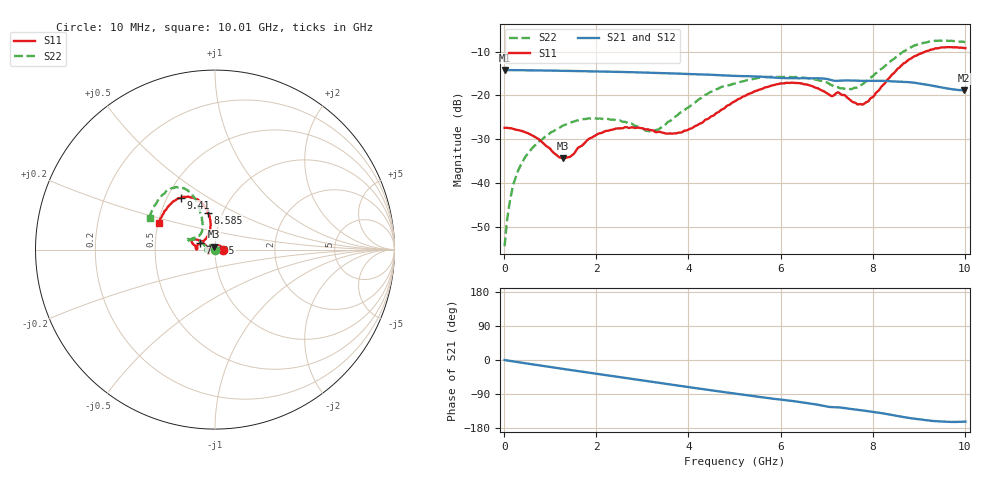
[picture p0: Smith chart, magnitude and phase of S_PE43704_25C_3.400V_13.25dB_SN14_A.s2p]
! Device ID: PE43704
! Dir: z:\PE43704\PE43704_Char_1_20130516\PE43704\AMB\3p400V\13p25dB
! Serial: 14
! Insertion: A
! Impedance: 50 ohm
! Temp: Amb
! VDD: 3.400V
! Attenuation Step: 13.25dB
! IDD: 1.140195e-01mA
#  Hz  S  RI  R  50
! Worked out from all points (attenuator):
!   401 points, 10 MHz to 10.01 GHz, reference 50 ohm
!   highest |S21| = -14.22 dB at 10 MHz (marker M1); lowest = -18.9 dB at 9.985 GHz (marker M2)
!   lowest |S11| = -34.4 dB at 1.285 GHz (marker M3), VSWR 1.04, Z = 49.2 + j1.69 ohm
!   |S11| at or under -10 dB: start of sweep to 9.14 GHz
!   |S22| runs from -54.5 to -7.5 dB; largest |S21 - S12| = 0.0017
!   S11 on the Smith chart (normalised r, x): 10 MHz: 1.09, +0.00; 7.485 GHz: 0.84, +0.06; 8.585 GHz: 0.85, +0.37; 9.41 GHz: 0.59, +0.38; 10.01 GHz: 0.50, +0.17
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1e7  0.0425 0.000286  0.1946 -0.000713  0.1947 -0.00069  0.00183 0.000487
1.6e8  0.0415 0.00618  0.1938 -0.0105  0.1938 -0.0105  0.00161 0.00748
3.6e8  0.037 0.0137  0.1924 -0.023  0.1922 -0.0232  -0.00208 0.0158
7.35e8  0.0222 0.0231  0.187 -0.0454  0.187 -0.0454  -0.0147 0.025
1.285e9  -0.00815 0.0172  0.1747 -0.0764  0.1746 -0.0763  -0.0411 0.0192
1.685e9  -0.0263 0.00321  0.1624 -0.0968  0.1625 -0.0967  -0.0531 0.00531
2.01e9  -0.0346 -0.00853  0.1505 -0.1119  0.1506 -0.1117  -0.0538 -0.00518
2.435e9  -0.0364 -0.0204  0.133 -0.1292  0.1331 -0.1292  -0.0504 -0.0113
3.11e9  -0.0336 -0.0234  0.1013 -0.1507  0.1016 -0.1506  -0.0391 -0.00169
3.36e9  -0.0334 -0.0188  0.0886 -0.1565  0.0888 -0.1564  -0.0405 0.00649
4.01e9  -0.0407 0.00406  0.0548 -0.1663  0.055 -0.1662  -0.0671 0.0303
4.46e9  -0.051 0.022  0.0315 -0.1693  0.0317 -0.1694  -0.0944 0.0528
5.01e9  -0.0741 0.0426  0.00461 -0.1666  0.00472 -0.1668  -0.1257 0.0542
5.96e9  -0.122 0.0575  -0.038 -0.1537  -0.0374 -0.1539  -0.1538 0.0512
6.685e9  -0.1236 0.0321  -0.0677 -0.1412  -0.0678 -0.1411  -0.1448 0.0514
7.485e9  -0.0835 0.0359  -0.0922 -0.1155  -0.0921 -0.1157  -0.0844 0.0836
7.835e9  -0.0461 0.068  -0.102 -0.1056  -0.1019 -0.1058  -0.0697 0.124
8.36e9  -0.0256 0.1563  -0.1171 -0.0855  -0.1169 -0.0859  -0.0852 0.2217
8.585e9  -0.04 0.2051  -0.1218 -0.0743  -0.1215 -0.0745  -0.1071 0.2726
9.41e9  -0.1891 0.288  -0.1193 -0.0395  -0.1193 -0.0388  -0.2565 0.3317
9.985e9  -0.3075 0.1593  -0.1088 -0.0339  -0.1089 -0.0341  -0.3607 0.1856
1.001e10  -0.3125 0.1493  -0.1088 -0.034  -0.1094 -0.0346  -0.3646 0.1775
